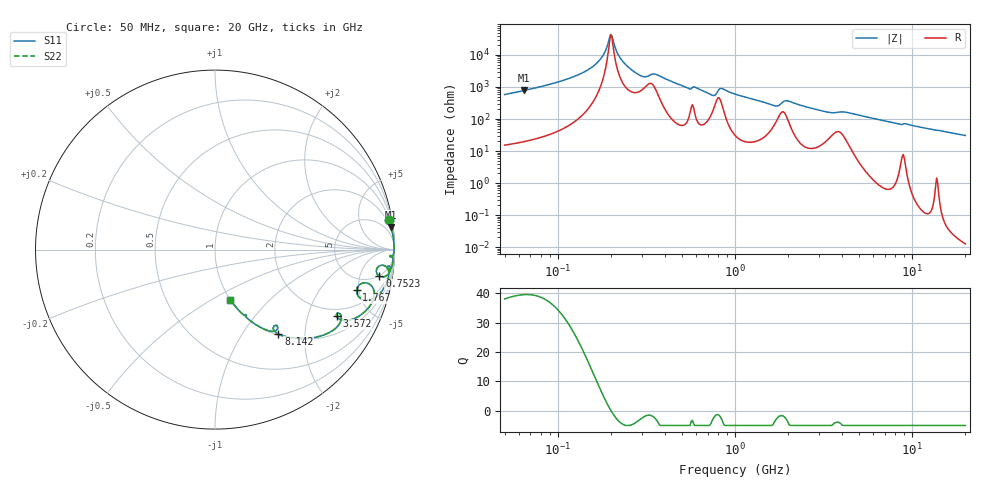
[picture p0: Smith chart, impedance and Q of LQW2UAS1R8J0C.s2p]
!Murata Part Number: LQW2UAS1R8J0C
!These Parameters are Measured in Series Mode Connection
!  o--[Z]--o
!Port1  Port2
!  o-------o
!Freq. Start=50[MHz] Stop=20[GHz], 401[Steps]
# Hz S RI R 50
!Freq.(Hz) S11(Real) S11(Imag) S21(Real) S21(Imag) S12(Real) S12(Imag) S22(Real) S22(Imag)
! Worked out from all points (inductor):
!   401 points, 50 MHz to 20 GHz, reference 50 ohm
!   read as one part in series: L = 1.72 uH near 51.52 MHz
!   highest Q = 39.5 at 64.5 MHz (marker M1), where L = 1.92 uH
!   self-resonance near 198.4 MHz
!   S11 on the Smith chart (normalised r, x): 50 MHz: 1, +12; 752.3 MHz: 5, -10; 1.767 GHz: 3.39, -4.72; 3.572 GHz: 1.66, -3.07; 8.142 GHz: 1.02, -1.47; 20 GHz: 1.00, -0.61
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5e7  0.967 0.1659  0.033 -0.1659  0.033 -0.1659  0.967 0.1659
6.449968e7  0.9807 0.1254  0.0193 -0.1254  0.0193 -0.1254  0.9807 0.1254
1.364002e8  0.9969 0.0367  0.00309 -0.0367  0.00309 -0.0367  0.9969 0.0367
1.733395e8  0.998 0.0136  0.00204 -0.0136  0.00204 -0.0136  0.998 0.0136
1.983553e8  0.9978 0.000595  0.00221 -0.000595  0.00221 -0.000595  0.9978 0.000595
2.043874e8  0.9977 -0.00235  0.00235 0.00235  0.00235 0.00235  0.9977 -0.00235
2.269813e8  0.9967 -0.013  0.00328 0.013  0.00328 0.013  0.9967 -0.013
2.597386e8  0.9934 -0.0278  0.00659 0.0278  0.00659 0.0278  0.9934 -0.0278
3.017088e8  0.9796 -0.0416  0.0204 0.0416  0.0204 0.0416  0.9796 -0.0416
3.721004e8  0.9887 -0.0423  0.0113 0.0423  0.0113 0.0423  0.9887 -0.0423
5.411141e8  0.9786 -0.104  0.0214 0.104  0.0214 0.104  0.9786 -0.104
7.523192e8  0.9157 -0.1484  0.0843 0.1484  0.0843 0.1484  0.9157 -0.1484
8.354841e8  0.9519 -0.0939  0.0481 0.0939  0.0481 0.0939  0.9519 -0.0939
1e9  0.9652 -0.1593  0.0348 0.1593  0.0348 0.1593  0.9652 -0.1593
1.766834e9  0.7888 -0.2271  0.2112 0.2271  0.2112 0.2271  0.7888 -0.2271
1.962148e9  0.8763 -0.2073  0.1237 0.2073  0.1237 0.2073  0.8763 -0.2073
2.728004e9  0.8077 -0.367  0.1923 0.367  0.1923 0.367  0.8077 -0.367
3.572216e9  0.6777 -0.372  0.3223 0.372  0.3223 0.372  0.6777 -0.372
4.472136e9  0.6852 -0.4248  0.3148 0.4248  0.3148 0.4248  0.6852 -0.4248
7.442007e9  0.4036 -0.4868  0.5964 0.4868  0.5964 0.4868  0.4036 -0.4868
8.141811e9  0.3531 -0.4705  0.6469 0.4705  0.6469 0.4705  0.3531 -0.4705
2e10  0.0855 -0.2794  0.9145 0.2794  0.9145 0.2794  0.0855 -0.2794
